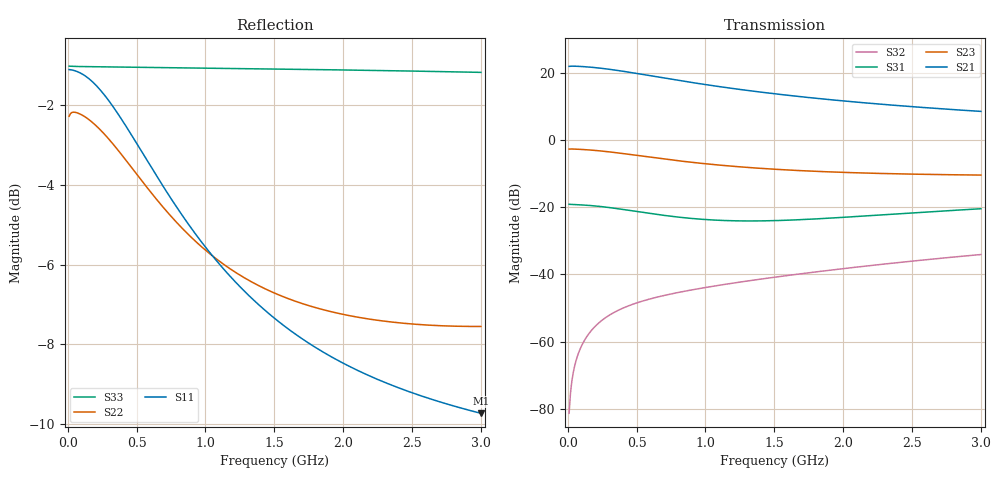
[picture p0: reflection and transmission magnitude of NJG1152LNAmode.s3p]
! Created Fri Sep 07 18:22:42 2012
# hz S ma R 50
! 3 Port Network Data Port1:RFIN  Port2:RFOUT  Port3:RFOUT2
! freq  magS11  angS11  magS12  angS12  magS13  angS13
!  magS21  angS21
!  magS22  angS22  magS23  angS23
!  magS31  angS31  magS32  angS32
!  magS33  angS33
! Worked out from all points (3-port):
!   300 points, 10 MHz to 3 GHz, reference 50 ohm
!   strongest paths, dB at 10 MHz, 760 MHz, 1.51 GHz, 2.26 GHz, 3 GHz:
!     S21: 21.9, 18.0, 13.7, 10.7, 8.5
!     S23: -2.7, -6.0, -8.7, -9.9, -10.4
!     S31: -19.1, -22.7, -24.0, -22.3, -20.5
!     S32: -81.3, -45.7, -40.8, -37.1, -34.1
!   lowest |S11| = -9.7 dB at 3 GHz (marker M1), VSWR 1.97, Z = 25.8 - j5.35 ohm
!   |S11| at or under -10 dB: nowhere
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1e7  0.8801 -1.3  0.0009981 73.6  0.1105 -0.5
     12.45 179.3  0.7691 0.0  0.732 179.5
     0.1105 -0.6  8.601e-05 78.6  0.8888 -0.1
8e7  0.8733 -10.4  0.00774 83.1  0.1089 -3.1
     12.44 171.3  0.7754 -4.8  0.7271 173.4
     0.1087 -3.9  0.0006922 85.7  0.8879 -0.7
2.5e8  0.8244 -31.4  0.02307 74.5  0.1037 -8.1
       11.61 153.5  0.7355 -14.6  0.6832 160.8
       0.1018 -10.6  0.002091 82.3  0.8871 -2.1
3.6e8  0.7767 -43.7  0.03157 69.3  0.09878 -10.3
       10.83 143.4  0.6993 -19.6  0.6438 153.9
       0.09523 -13.5  0.002885 80.2  0.8865 -3.0
4.9e8  0.716 -56.7  0.04011 64.2  0.0927 -11.7
       9.844 132.9  0.6544 -24.4  0.5944 147.1
       0.08702 -15.2  0.003709 78.8  0.8858 -4.0
7e8  0.6255 -74.5  0.05125 58.4  0.08409 -11.6
     8.348 118.9  0.5896 -29.9  0.5212 138.7
     0.07557 -14.2  0.004867 78.6  0.8848 -5.6
9.3e8  0.547 -90.3  0.06128 54.3  0.07737 -9.3
       7.01 106.8  0.5357 -33.8  0.4585 132.3
       0.06722 -9.4  0.006039 80.1  0.8838 -7.4
1.51e9  0.4282 -119.5  0.08339 47.9  0.07064 -0.1
        4.845 84.5  0.4611 -40.0  0.3663 122.0
        0.06325 7.6  0.009143 86.1  0.8814 -12.0
2.12e9  0.3684 -141.0  0.106 42.3  0.07243 8.8
        3.621 66.9  0.4303 -46.0  0.3239 113.7
        0.07321 19.3  0.01301 91.2  0.8785 -16.8
3e9  0.3264 -163.5  0.1383 33.0  0.08239 17.0
     2.661 45.5  0.4194 -56.5  0.3006 101.4
     0.0949 24.2  0.01978 95.2  0.873 -23.7
